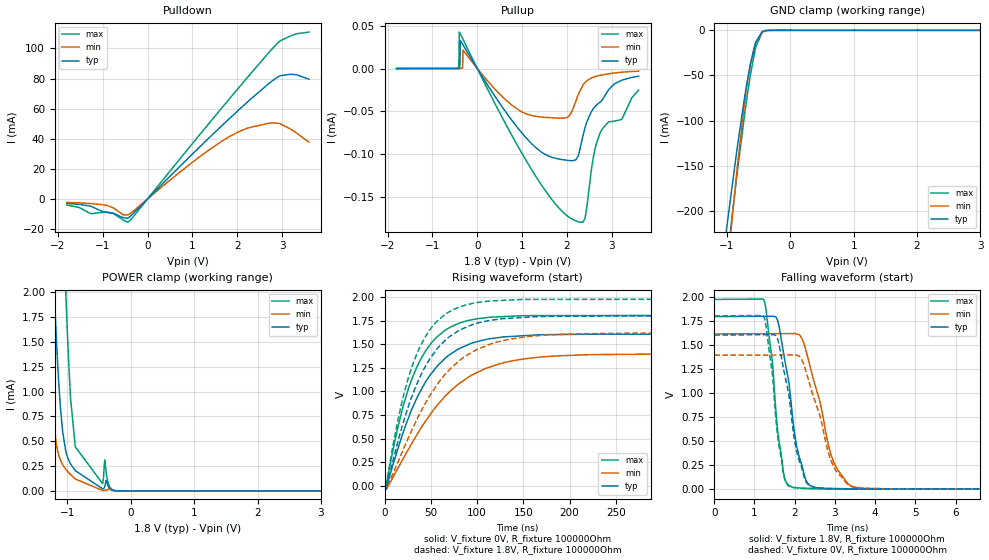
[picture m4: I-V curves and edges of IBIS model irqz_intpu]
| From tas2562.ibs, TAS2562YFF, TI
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|   irqz_intpu Model
[Model]   irqz_intpu
Model_type   3-state
Polarity   Non-Inverting
Vmeas = 0.9
Vref = 0
Cref = 2pF
Rref = 100000
|   typ   min   max
C_comp   2.003pF   1.966pF   2.088pF
| Where Nom  PVT is Nominal Process, 1.8V, 25C
|   Fast PVT is Strong Process,  1.98V, -40C
|   Slow PVT is Weak Process,   1.62V, 150C
[Voltage Range]   1.8   1.62   1.98
|Junction Temperature
[Temperature Range]   25   150   -40
[Pullup Reference]   1.8   1.62   1.98
[Pulldown Reference]   0   0   0
[Power Clamp Reference]   1.8   1.62   1.98
[GND Clamp Reference]   0   0   0
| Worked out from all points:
|   slope of the pulldown table from 0 to 0.27 V, typ, clamps not added: 33.2 ohm
|   slope of the pullup table from 0 to 0.27 V, typ, clamps not added: 12.1 kohm
|   GND clamp passes 1 mA (typ) near -0.43 V on its own axis
|   POWER clamp passes 1 mA (typ) near -1.13 V on its own axis
|   falling waveform, V_fixture 1.8V, R_fixture 100000Ohm: 20-80 % time 382ps typ, 560ps min, 285ps max; typ from 1.8 V to 0.001 V
|   rising waveform, V_fixture 0V, R_fixture 100000Ohm: 20-80 % time 46.4ns typ, 66ns min, 36.7ns max; typ from 0 V to 1.61 V
|   rising waveform, V_fixture 1.8V, R_fixture 100000Ohm: 20-80 % time 44.4ns typ, 59.7ns min, 35.7ns max; typ from 0.001 V to 1.8 V
|   falling waveform, V_fixture 0V, R_fixture 100000Ohm: 20-80 % time 385ps typ, 565ps min, 287ps max; typ from 1.61 V to 0 V
[Pulldown]
|   Voltage   I(typ)   I(min)   I(max)
-1.8V     -2.957mA   -2.3mA     -4.034mA
-1.525V   -3.634mA   -2.61mA    -5.679mA
-1.26V    -4.892mA   -3.1mA     -9.788mA
-925.2mV  -8.723mA   -4.215mA   -8.896mA
-547.2mV  -12.42mA   -10.54mA   -13.89mA
-412.2mV  -12.21mA   -10.16mA   -14.9mA
1.219V    36.12mA    29.23mA    44.65mA
2.126V    61.6mA     45.81mA    77.08mA
2.687V    76.17mA    50.19mA    96.55mA
2.957V    81.7mA     49.87mA    104.9mA
3.276V    82.66mA    44.75mA    109.2mA
3.6V      79.58mA    37.74mA    110.8mA
[GND Clamp]
|   Voltage   I(typ)   I(min)   I(max)
-1.8V     -830.2mA   -917.2mA   -810.3mA
-1.017V   -226mA     -280.9mA   -265mA
-849.6mV  -136.2mA   -160.2mA   -164.9mA
-725.4mV  -76.2mA    -82.49mA   -95.68mA
-676.8mV  -55.51mA   -57.51mA   -71.17mA
-628.2mV  -37.22mA   -36.99mA   -48.97mA
-558mV    -16.53mA   -16.23mA   -22.83mA
-541.8mV  -12.94mA   -12.9mA    -18.1mA
-439.2mV  -1.277mA   -1.972mA   -1.711mA
-385.2mV  -225.2uA   -567.9uA   -219.6uA
-261mV    -2.2uA     -22.37uA   -652.9nA
3.6V      0A         0A         0A
[Pullup]
|   Voltage   I(typ)   I(min)   I(max)
-1.8V     46pA       120pA      108pA
-444.6mV  34.89nA    353pA      220.3nA
-412.2mV  102.7nA    53.47nA    3.684uA
-401.4mV  198.2nA    39.95nA    42.43uA
-379.8mV  32.79uA    23.09nA    40.36uA
-320.4mV  27.68uA    21.55uA    34.25uA
1.229V    -88.4uA    -54.93uA   -119.2uA
2.007V    -106.9uA   -56.87uA   -171.5uA
2.272V    -98.2uA    -28.11uA   -178.9uA
2.407V    -68.61uA   -16.16uA   -173.2uA
2.741V    -38.97uA   -7.887uA   -75.04uA
3.6V      -8.897uA   -3.074uA   -25.19uA
[POWER Clamp]
|   Voltage   I(typ)   I(min)   I(max)
-1.8V     15.69mA    11.82mA    24.27mA
-1.352V   4.592mA    2.132mA    9.4mA
-1.249V   2.668mA    900.4uA    6.926mA
-1.152V   1.249mA    396.7uA    4.653mA
-1.082V   632.3uA    271.2uA    3.097mA
-1.022V   390.1uA    214.6uA    1.943mA
-952.2mV  272.5uA    165.5uA    941.7uA
-876.6mV  204.9uA    120.4uA    444.5uA
-444.6mV  21.3uA     4.377uA    72.73uA
-412.2mV  43.5uA     7.407uA    311.6uA
-255.6mV  1.618uA    6.067uA    2.772uA
3.6V      0A         0A         0A
[Ramp]
R_load = 100000
|   typ   min   max
dV/dt_r   0.964508/4.64163e-08   0.838406/6.57787e-08   1.08441/3.67484e-08
dV/dt_f   1.07963/3.83336e-10   0.971423/5.59471e-10   1.18704/2.86593e-10
[Falling Waveform]
V_fixture = 1.8V
V_fixture_min = 1.62V
V_fixture_max = 1.98V
R_fixture = 100000Ohm
C_fixture = 0F
|   Time   V(typ)   V(min)   V(max)
0s        1.8V       1.62V      1.979V
1.233ns   1.803V     1.622V     1.975V
1.446ns   1.804V     1.622V     1.327V
1.538ns   1.794V     1.622V     787.2mV
1.772ns   1.304V     1.623V     88.24mV
2.034ns   485.4mV    1.622V     15.56mV
2.22ns    180.1mV    1.529V     8.788mV
2.956ns   6.805mV    297.7mV    2.693mV
3.717ns   2.734mV    9.181mV    2.69mV
100ns     595.3uV    637.6uV    534.6uV
[Rising Waveform]
V_fixture = 0V
V_fixture_min = 0V
V_fixture_max = 0V
R_fixture = 100000Ohm
C_fixture = 0F
|   Time   V(typ)   V(min)   V(max)
0s        11.93nV    16.41nV    37.25nV
1.295ns   1.748mV    623.4uV    -35.23mV
2.219ns   -12.71mV   -33.2mV    20.16mV
18.91ns   528.8mV    265.1mV    797.1mV
34.55ns   921mV      533.1mV    1.251V
53.34ns   1.224V     809.2mV    1.544V
80.26ns   1.452V     1.08V      1.722V
124.9ns   1.573V     1.294V     1.792V
176.8ns   1.602V     1.371V     1.804V
500ns     1.608V     1.397V     1.807V
[Rising Waveform]
V_fixture = 1.8V
V_fixture_min = 1.62V
V_fixture_max = 1.98V
R_fixture = 100000Ohm
C_fixture = 0F
|   Time   V(typ)   V(min)   V(max)
0s        595.3uV    637.6uV    534.6uV
1.295ns   2.344mV    1.261mV    -34.21mV
2.219ns   -7.529mV   -31.57mV   26.73mV
18.91ns   625.1mV    353.1mV    892mV
34.55ns   1.071V     694.9mV    1.389V
53.34ns   1.405V     1.02V      1.708V
80.26ns   1.646V     1.321V     1.893V
114ns     1.753V     1.501V     1.959V
167.5ns   1.793V     1.593V     1.975V
500ns     1.8V       1.62V      1.979V
[Falling Waveform]
|Gnd
V_fixture = 0V
V_fixture_min = 0V
V_fixture_max = 0V
R_fixture = 100000Ohm
C_fixture = 0F
|   Time   V(typ)   V(min)   V(max)
0s        1.608V     1.397V     1.807V
1.233ns   1.611V     1.399V     1.803V
1.443ns   1.611V     1.399V     1.214V
1.533ns   1.604V     1.399V     727.6mV
1.772ns   1.153V     1.4V       78.42mV
2.034ns   424.1mV    1.398V     13.81mV
2.22ns    154.4mV    1.309V     7.629mV
2.956ns   5.61mV     246.6mV    1.999mV
3.717ns   1.947mV    7.393mV    1.996mV
100ns     11.35nV    -293.8nV   37.72nV
